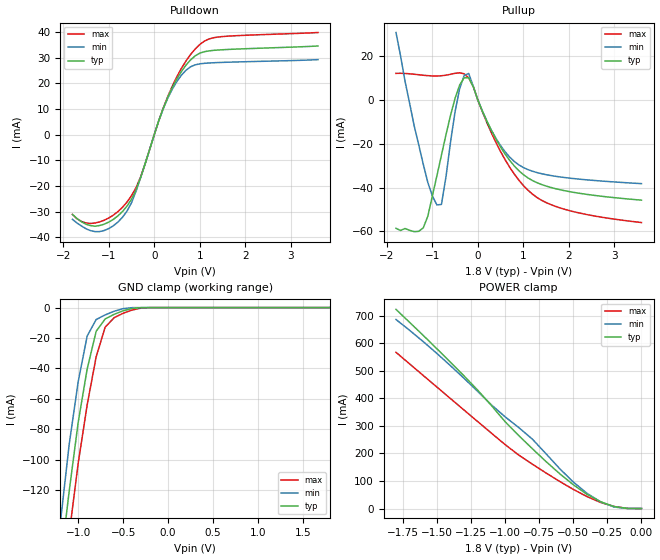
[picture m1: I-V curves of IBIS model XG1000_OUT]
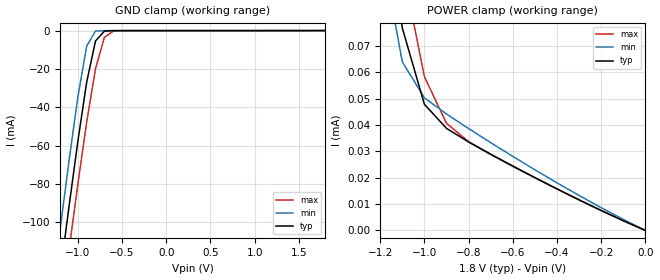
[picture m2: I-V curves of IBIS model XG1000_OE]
|   IBIS File xg1kca-e.ibs
|   Epson Toyocom Corporation , 2005
[IBIS Ver]   2.1
[Comment Char]   |_char
[File name]   xg1kca-e.ibs
[File Rev]   2.0
[Date]   2006/12/26
[Source]
[Notes]
[Disclaimer]
This information is for modeling purposes only, and is not guaranteed.
Property of Epson Toyocom Corp.,
unauthorized reproduction and/or distribution is strictly prohibited.
[Copyright]
Copyright 2005, Epson Toyocom Corp.
|   Component XG-1000CA_E
[Component]   XG-1000CA_E
[Manufacturer]   Epson Toyocom Corp.
[Package]
| variable   typ   min   max
R_pkg   0.878   NA   NA
L_pkg   2.13nH   NA   NA
C_pkg   3.21pF   NA   NA
[Pin]signal_name   model_name   R_pin   L_pin   C_pin
1   oe   XG1000_OE   NA   NA   NA
2   vss   GND   NA   NA   NA
3   out   XG1000_OUT   NA   NA   NA
4   vdd   POWER   NA   NA   NA
| Models and submodels in the file (2): XG1000_OUT (3-state), XG1000_OE (Input)
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|   Model XG1000_OUT
[Model]   XG1000_OUT
Model_type 3-state
Enable Active-High
Polarity Inverting
C_comp   3p   2.5p   3.5p
[Temperature Range] 25   -40   85
[Voltage Range]   1.8   1.7   1.9
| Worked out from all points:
|   slope of the pulldown table from 0 to 0.27 V, typ, clamps not added: 20.2 ohm
|   slope of the pullup table from 0 to 0.27 V, typ, clamps not added: 21.3 ohm
|   GND clamp passes 1 mA (typ) near -0.43 V on its own axis
|   POWER clamp passes 1 mA (typ) near -0.11 V on its own axis
[Pullup]
-1.8V     -58.6mA    30.78mA    12.15mA
-1.2V     -58.37mA   -29.37mA   11.29mA
-900mV    -34.61mA   -47.93mA   10.95mA
-800mV    -25.19mA   -47.69mA   11.05mA
-500mV    783.9uA    -5.333mA   12.17mA
-400mV    6.792mA    5.15mA     12.41mA
-200mV    10.14mA    12.09mA    10.04mA
100mV     -5.021mA   -5.07mA    -5.354mA
500mV     -21.48mA   -20.82mA   -23.52mA
1.2V      -36.76mA   -32.52mA   -42.97mA
2V        -41.78mA   -35.64mA   -50.43mA
3.6V      -45.74mA   -38.2mA    -55.96mA
[Pulldown]
-1.8V     -31.08mA   -33mA      -31.09mA
-1.5V     -34.94mA   -36.69mA   -34.45mA
-1.2V     -35.41mA   -37.78mA   -33.99mA
-900mV    -33.02mA   -35.51mA   -31.37mA
-600mV    -27.86mA   -29.81mA   -26.28mA
-300mV    -16.69mA   -16.78mA   -16.47mA
100mV     5.458mA    5.449mA    5.482mA
300mV     14.65mA    14.3mA     14.97mA
600mV     24.68mA    23.22mA    25.91mA
800mV     29.14mA    26.45mA    31.25mA
1.3V      32.83mA    28.01mA    37.74mA
3.6V      34.54mA    29.23mA    39.78mA
[GND Clamp]
-1.8V     -474.8mA   -466.9mA   -489.5mA
-1.2V     -170.3mA   -142.5mA   -196.7mA
-1.1V     -120.7mA   -89.99mA   -148.9mA
-1V       -75.55mA   -48.78mA   -102.4mA
-900mV    -40.37mA   -18.72mA   -63.95mA
-800mV    -15.58mA   -7.854mA   -32.35mA
-700mV    -7.457mA   -4.83mA    -12.88mA
-600mV    -4.429mA   -2.41mA    -6.64mA
-500mV    -2.099mA   -692uA     -3.747mA
-400mV    -554.4uA   -62.41uA   -1.607mA
-300mV    -51.39uA   -1.685uA   -355.2uA
1.8V      2.251nA    240.6nA    -175.1nA
[POWER Clamp]
-1.8V     722.5mA    685.8mA    566.8mA
-1.6V     628mA      605.5mA    482.7mA
-1.3V     480.6mA    472mA      356.9mA
-1.2V     428.9mA    424.6mA    315.1mA
-1V       315mA      332.7mA    231.9mA
-800mV    217mA      251.7mA    160.9mA
-500mV    86.3mA     96.2mA     69.45mA
-400mV    51.62mA    55.26mA    43.48mA
-300mV    24.52mA    24.33mA    22.06mA
-200mV    6.958mA    5.264mA    7.215mA
-100mV    33.06uA    240.6nA    287.9uA
0V        2.251nA    6.729pA    145.5nA
[Ramp]
R_load=50
dV/dt_r   7.282E-1/1.060E-10   6.811E-1/1.266E-10   7.934E-1/1.066E-10
dV/dt_f   7.286E-1/1.233E-10   6.772E-1/9.473E-11   7.789E-1/1.103E-10
|   Model XG1000_OE
[Model]   XG1000_OE
Model_type Input
Vinh=1.19
Vinl=0.51
C_comp   3p   2.5p   3.5p
[Temperature Range] 25   -40   85
[Voltage Range]   1.8   1.7   1.9
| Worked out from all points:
|   GND clamp passes 1 mA (typ) near -0.71 V on its own axis
[GND Clamp]
-1.8V     -349.1mA   -326.5mA   -371.1mA
-1.3V     -163.4mA   -139.8mA   -186.1mA
-1.2V     -127.3mA   -103.5mA   -150mA
-1.1V     -91.88mA   -68.12mA   -114.6mA
-1V       -57.86mA   -34.77mA   -80.22mA
-900mV    -26.93mA   -8.079mA   -47.8mA
-800mV    -5.398mA   -245.8uA   -19.85mA
-700mV    -298.7uA   -24.24uA   -3.581mA
-600mV    -29.34uA   -22.68uA   -298.2uA
1.8V      1.798pA    4.192uA    -3.481uA
[POWER Clamp]
-1.8V     658.2uA    635uA      684.8uA
-1.2V     135.3uA    109.7uA    164.7uA
-1.1V     76.84uA    63.97uA    100.5uA
-1V       47.87uA    50.32uA    58.33uA
-900mV    38.73uA    44.18uA    40.67uA
-800mV    33.58uA    38.66uA    33.66uA
-700mV    28.94uA    33.31uA    28.8uA
-500mV    20.06uA    23.02uA    19.98uA
-300mV    11.6uA     13.27uA    11.59uA
-100mV    3.686uA    4.192uA    3.698uA
0V        1.666pA    1.414pA    2.775pA
